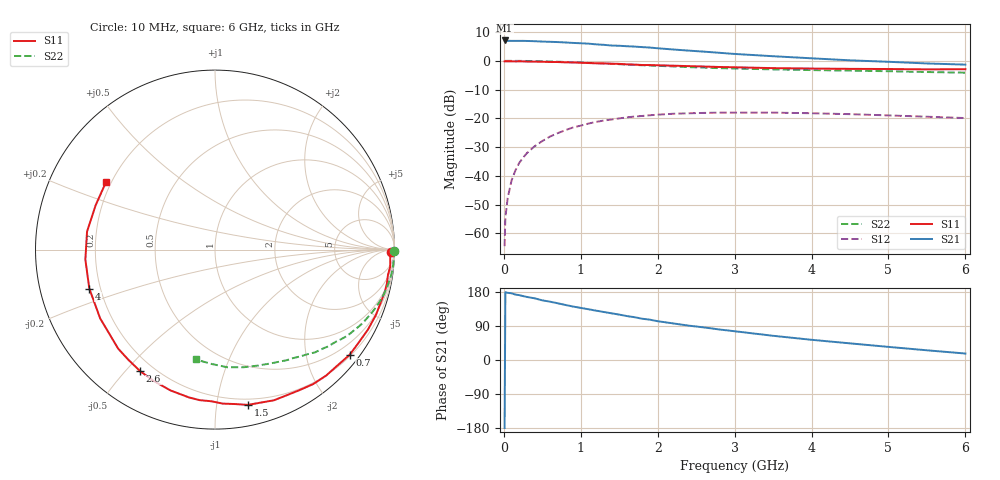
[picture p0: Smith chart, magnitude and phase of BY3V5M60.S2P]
! SIEMENS Small Signal Semiconductors
! BFY420
! Si NPN RF SIEGET Grounded Emitter Transistor in MICRO-X
! VCE = 3.5 V  IC = 0.6 mA
! Common Emitter S-Parameters:  October  1996
# GHz  S  MA  R  50
!  f  S11  S21  S12  S22
! GHz  MAG  ANG  MAG  ANG  MAG  ANG  MAG  ANG
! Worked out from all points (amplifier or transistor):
!   36 points, 10 MHz to 6 GHz, reference 50 ohm
!   highest |S21| = 7.1 dB at 10 MHz (marker M1)
!   |S21| within 3 dB of that: start of sweep to 2.134 GHz
!   unconditionally stable (mu >= 1): 4.723 GHz to end of sweep
!   at 250 MHz: K = 0.05, MSG = 20.3 dB, |S12| = -33.7 dB
!   at 1.4 GHz: K = 0.16, MSG = 12.9 dB, |S12| = -20.4 dB
!   at 6 GHz: K = 1.42, MAG = 5.4 dB, |S12| = -19.9 dB
!   S11 on the Smith chart (normalised r, x): 10 MHz: 71, -42; 700 MHz: 0.23, -2.89; 1.5 GHz: 0.15, -1.22; 2.6 GHz: 0.15, -0.55; 4 GHz: 0.16, -0.15; 6 GHz: 0.18, +0.27
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0.01  0.9794 -0.7  2.257 -179.3  0.0006 92.1  0.9999 -0.3
0.02  0.9761 -1.2  2.247 178.8  0.0019 87.7  0.9955 -0.5
0.05  0.9771 -2.8  2.221 177.3  0.0041 84.8  0.9982 -1.3
0.1  0.9809 -5.7  2.22 176.0  0.0083 87.7  0.9978 -2.5
0.15  0.974 -8.2  2.218 172.7  0.0124 83.9  0.9967 -3.8
0.2  0.9762 -11.1  2.219 171.2  0.0168 84.5  0.9966 -4.9
0.25  0.9751 -13.8  2.221 168.7  0.0207 80.2  0.9945 -6.2
0.4  0.9678 -22.1  2.191 162.8  0.0327 76.4  0.9878 -10.0
0.5  0.9617 -27.6  2.159 157.4  0.0403 73.2  0.9808 -12.4
0.7  0.9519 -38.0  2.116 149.7  0.0552 66.9  0.9638 -17.2
0.9  0.936 -48.6  2.045 141.0  0.0694 59.9  0.9429 -21.7
1.1  0.9139 -58.8  1.985 133.9  0.0811 54.0  0.9205 -26.1
1.5  0.8844 -78.0  1.825 119.8  0.0998 42.6  0.8733 -33.9
1.8  0.8452 -91.4  1.729 108.9  0.11 35.1  0.8369 -39.1
2.2  0.823 -107.5  1.573 96.6  0.1201 26.3  0.7993 -45.7
2.6  0.7954 -121.6  1.443 86.0  0.1242 18.8  0.7614 -51.4
3  0.7716 -134.4  1.316 75.9  0.1256 12.5  0.7346 -57.0
3.5  0.7458 -149.1  1.201 63.9  0.1257 6.0  0.7085 -63.2
4  0.7331 -162.8  1.105 53.3  0.1226 0.9  0.6893 -69.6
4.5  0.7244 -175.6  1.019 43.9  0.1181 -3.2  0.6747 -76.3
5.5  0.7094 159.7  0.899 25.6  0.1067 -6.8  0.6379 -91.5
6  0.7141 148.4  0.858 17.1  0.1011 -6.1  0.6215 -100.0
